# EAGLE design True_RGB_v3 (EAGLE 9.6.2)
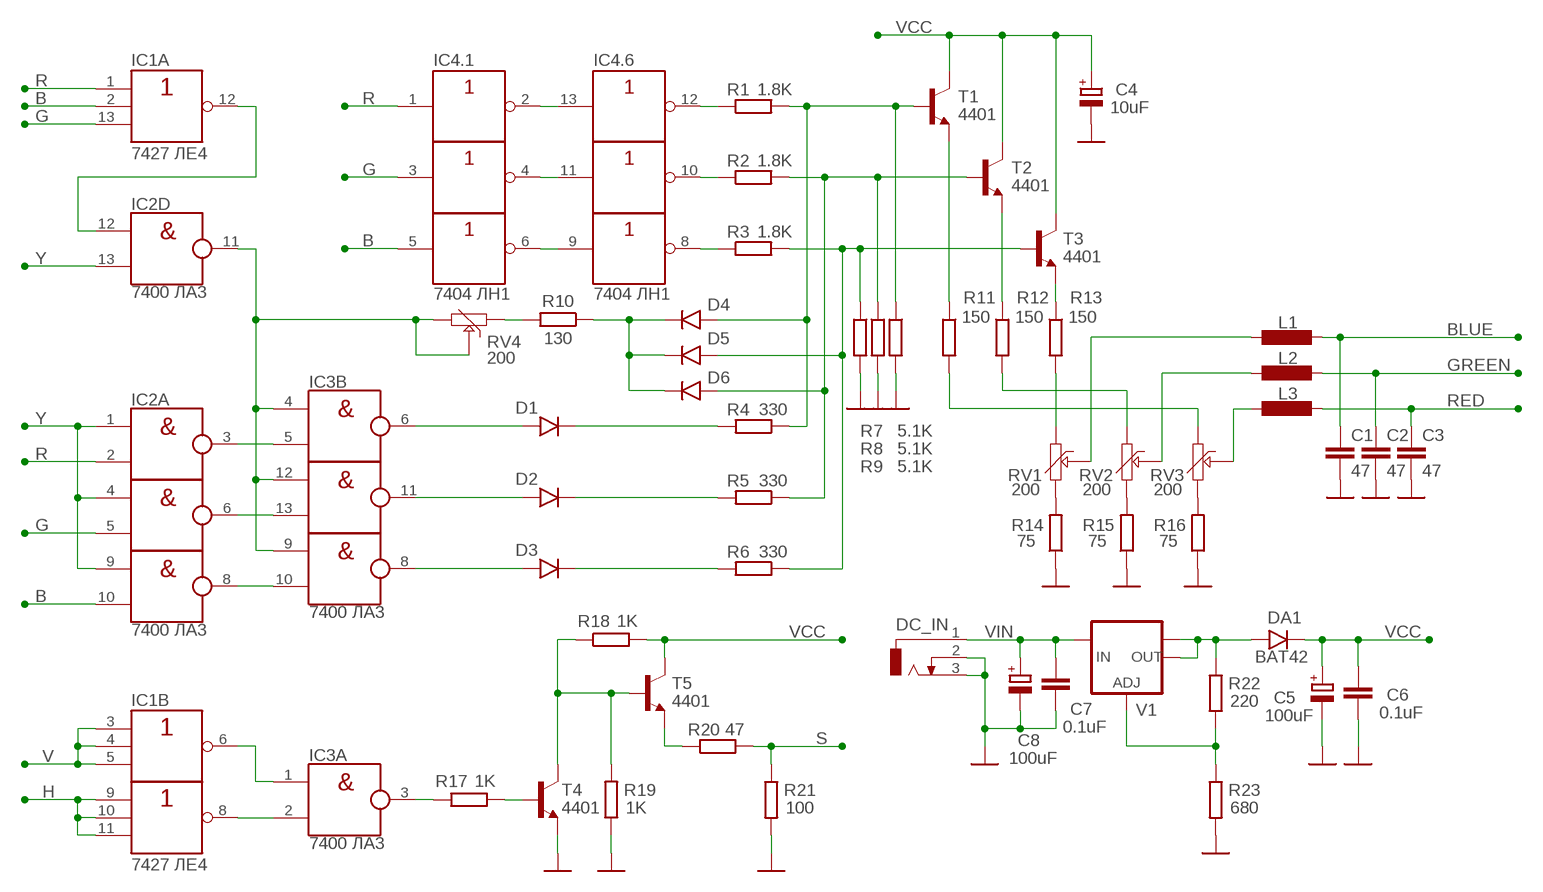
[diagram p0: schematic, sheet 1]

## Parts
C1  47  C-EU050-024X044  [C050-024X044]
C2  47  C-EU050-024X044  [C050-024X044]
C3  47  C-EU050-024X044  [C050-024X044]
C4  10uF  CPOL-EUE2.5-6  [E2,5-6]
C5  100uF  CPOL-EUE2.5-6  [E2,5-6]
C6  0.1uF  C-EU050-024X044  [C050-024X044]
C7  0.1uF  C-EU050-024X044  [C050-024X044]
C8  100uF  CPOL-EUE2.5-6  [E2,5-6]
D1  1N4148AS  [D4148-2]
D2  1N4148AS  [D4148-2]
D3  1N4148AS  [D4148-2]
D4  1N4148AS  [D4148-2]
D5  1N4148AS  [D4148-2]
D6  1N4148AS  [D4148-2]
DA1  BAT42  1N4148AS  [D4148-2]
DC_IN  DCJ0202  [DCJ0202]
IC1  7427 ЛЕ4  74HC27N  [DIL14]
IC2  7400 ЛА3  74HC00N  [DIL14]
IC3  7400 ЛА3  74HC00N  [DIL14]
IC4  7404 ЛН1  74HC04N  [DIL14]
L1  0.56uH  L-EU0207/2V  [0207/2V]
L2  0.56uH  L-EU0207/2V  [0207/2V]
L3  0.56uH  L-EU0207/2V  [0207/2V]
R1  1.8K  R-EU_0207/2V  [0207/2V]
R2  1.8K  R-EU_0207/2V  [0207/2V]
R3  1.8K  R-EU_0207/2V  [0207/2V]
R4  330  R-EU_0207/2V  [0207/2V]
R5  330  R-EU_0207/2V  [0207/2V]
R6  330  R-EU_0207/2V  [0207/2V]
R7  5.1K  R-EU_0207/2V  [0207/2V]
R8  5.1K  R-EU_0207/2V  [0207/2V]
R9  5.1K  R-EU_0207/2V  [0207/2V]
R10  130  R-EU_0207/2V  [0207/2V]
R11  150  R-EU_0207/2V  [0207/2V]
R12  150  R-EU_0207/2V  [0207/2V]
R13  150  R-EU_0207/2V  [0207/2V]
R14  75  R-EU_0207/2V  [0207/2V]
R15  75  R-EU_0207/2V  [0207/2V]
R16  75  R-EU_0207/2V  [0207/2V]
R17  1K  R-EU_0207/2V  [0207/2V]
R18  1K  R-EU_0207/2V  [0207/2V]
R19  1K  R-EU_0207/2V  [0207/2V]
R20  47  R-EU_0207/2V  [0207/2V]
R21  100  R-EU_0207/2V  [0207/2V]
R22  220  R-EU_0207/2V  [0207/2V]
R23  680  R-EU_0207/2V  [0207/2V]
RV1  200  TRIM-6MM  [6MM]
RV2  200  TRIM-6MM  [6MM]
RV3  200  TRIM-6MM  [6MM]
RV4  200  TRIM-6MM  [6MM]
T1  4401  2N4401-NPN-TO92-EBC  [TO92-EBC]
T2  4401  2N4401-NPN-TO92-EBC  [TO92-EBC]
T3  4401  2N4401-NPN-TO92-EBC  [TO92-EBC]
T4  4401  2N4401-NPN-TO92-EBC  [TO92-EBC]
T5  4401  2N4401-NPN-TO92-EBC  [TO92-EBC]
V1  LM1117IMPX-ADJ  [SOT223]

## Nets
B: IC1.2(A:I1) IC2.10(C:I1) IC4.5(.3:I)
BLUE: C1.1 L1.1
G: IC1.13(A:I2) IC2.5(B:I1) IC4.3(.2:I)
GND: C1.2 C2.2 C3.2 C4.- C5.- C6.2 C7.2 C8.- DC_IN.2 DC_IN.3 R7.2 R8.2 R9.2 R14.1 R15.1 R16.1 R19.1 R21.2 R23.2 T4.E
GREEN: C2.1 L2.1
H: IC1.9(C:I0) IC1.10(C:I1) IC1.11(C:I2)
N$1: D3.C R6.2
N$2: D2.C R5.2
N$3: D1.C R4.2
N$4: L1.2 RV1.S
N$5: IC1.12(A:O) IC2.12(D:I0)
N$6: IC1.8(C:O) IC3.2(A:I1)
N$7: L2.2 RV2.S
N$8: D5.A R3.2 R6.1 R7.1 T3.B
N$9: D6.A R2.2 R5.1 R8.1 T2.B
N$10: D4.A R1.2 R4.1 R9.1 T1.B
N$11: L3.2 RV3.S
N$12: R14.2 RV1.A
N$13: R15.2 RV2.A
N$14: R16.2 RV3.A
N$15: R11.1 T1.E
N$16: R12.2 RV2.E
N$17: R11.2 RV3.E
N$18: R12.1 T2.E
N$19: IC2.3(A:O) IC3.5(B:I1)
N$20: IC2.6(B:O) IC3.13(D:I1)
N$21: IC2.8(C:O) IC3.10(C:I1)
N$22: D1.A IC3.6(B:O)
N$23: D2.A IC3.11(D:O)
N$24: D3.A IC3.8(C:O)
N$25: IC4.2(.1:O) IC4.13(.6:I)
N$26: IC4.4(.2:O) IC4.11(.5:I)
N$27: IC4.6(.3:O) IC4.9(.4:I)
N$28: IC4.12(.6:O) R1.1
N$29: IC4.10(.5:O) R2.1
N$30: IC4.8(.4:O) R3.1
N$31: IC3.3(A:O) R17.2
N$32: R22.2 R23.1 V1.1(ADJ)
N$33: IC1.6(B:O) IC3.1(A:I0)
N$34: R17.1 T4.B
N$35: DA1.A R22.1 V1.2(OUT) V1.TAB(OUT1)
N$36: D4.C D5.C D6.C R10.1
N$37: R10.2 RV4.E
N$38: IC2.11(D:O) IC3.4(B:I0) IC3.9(C:I0) IC3.12(D:I0) RV4.A RV4.S
N$39: R13.1 T3.E
N$40: R13.2 RV1.E
N$176: R20.1 T5.E
N$177: R18.1 R19.2 T4.C T5.B
R: IC1.1(A:I0) IC2.2(A:I1) IC4.1(.1:I)
RED: C3.1 L3.1
S: R20.2 R21.1
V: IC1.3(B:I0) IC1.4(B:I1) IC1.5(B:I2)
VCC: C4.+ C5.+ C6.1 DA1.C R18.2 T1.C T2.C T3.C T5.C
VIN: C7.1 C8.+ DC_IN.1 V1.3(IN)
Y: IC2.1(A:I0) IC2.4(B:I0) IC2.9(C:I0) IC2.13(D:I1)

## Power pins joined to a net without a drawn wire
GND: IC1.7(P:GND) IC2.7(P:GND) IC3.7(P:GND) IC4.7(P:GND)
VCC: IC1.14(P:VCC) IC2.14(P:VCC) IC3.14(P:VCC) IC4.14(P:VCC)

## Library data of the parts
C1-C3 C6 C7 = rcl:C-EU: CAPACITOR, European symbol; SPICEPREFIX: C
C4 C5 C8 = rcl:CPOL-EU: POLARIZED CAPACITOR, European symbol; SPICEPREFIX: C
D1-D6 DA1 = 27C322:1N4148
DC_IN = power_jack:DCJ0202: DC POWER JACK Source: DCJ0202.pdf; OC_FARNELL: unknown; OC_NEWARK: unknown
IC1 = 74xx-eu:74*27: Triple 3-input NOR gate
IC2 IC3 = 74xx-eu:74*00: Quad 2-input NAND gate
IC4 = 74xx-eu:74*04: Hex INVERTER
L1-L3 = rcl:L-EU: INDUCTOR, European symbol; SPICEPREFIX: L
R1-R23 = rcl:R-EU_: RESISTOR, European symbol; SPICEPREFIX: R
RV1-RV4 = 27C322:TRIM-6MM
T1-T5 = transistor-neu-to92:*-NPN-: NPN Transistror
V1 = lm1117:LM1117IMPX-ADJ

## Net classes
1 power: width 0.66 mm, clearance 0.254 mm

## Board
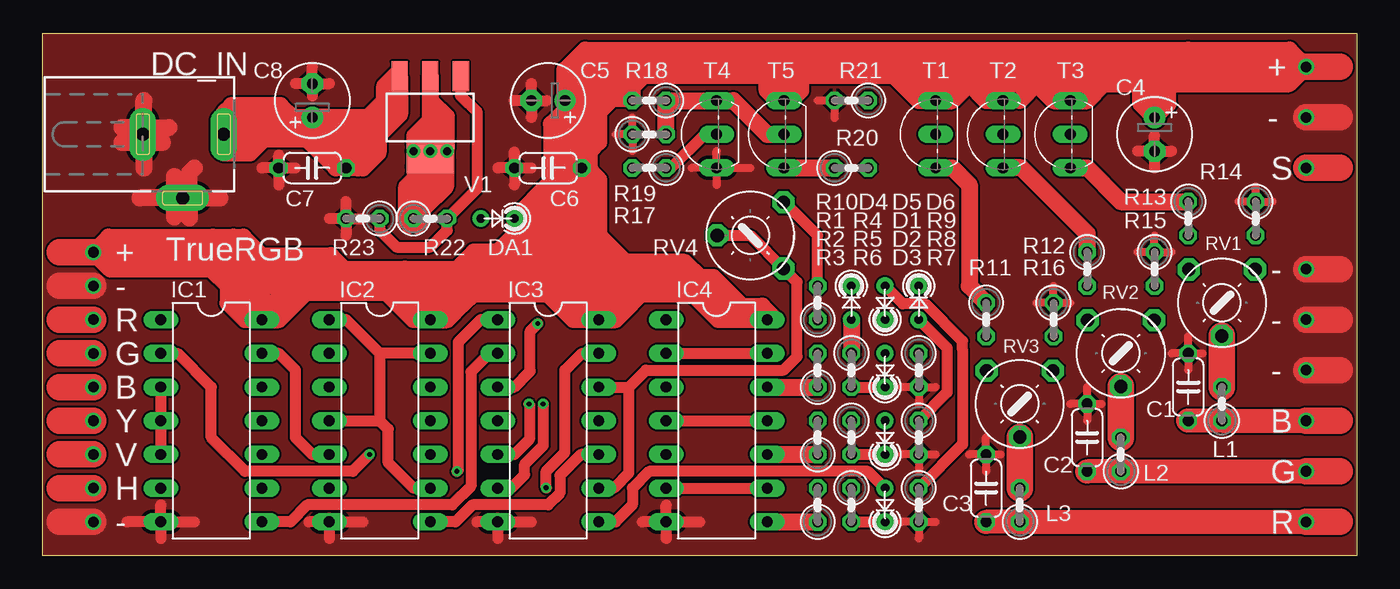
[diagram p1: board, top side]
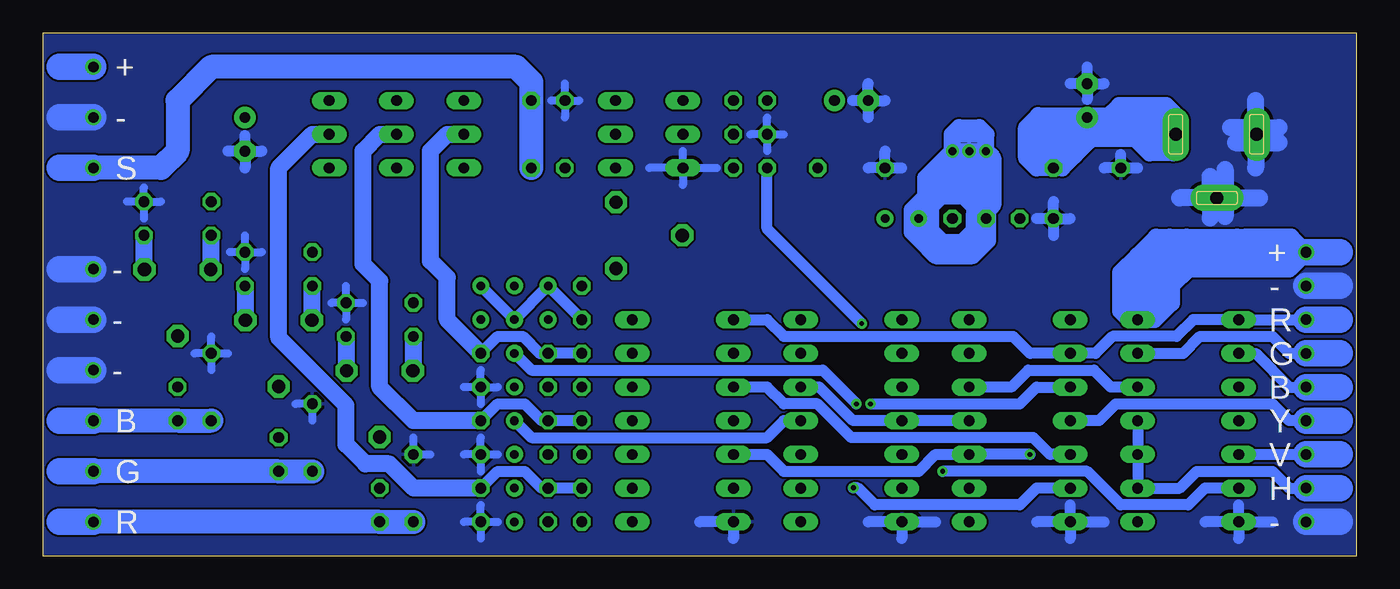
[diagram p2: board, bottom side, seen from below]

Size 99.06 x 39.37 mm. Coordinates in mm from the lower left corner, seen from the top.
Outline: 99.06,39.37 99.06,0 0,0 0,39.37 99.06,39.37
Copper layers (1*16): Top 0.035mm / dielectric 1.5mm / Bottom 0.035mm
Design rules "default *": minimum track width 6mil, minimum drill 0.35mm, track to track 6mil, track to pad 6mil, pad to pad 6mil, via to via 6mil, smd to smd 6mil, copper to edge 2mil, drill to drill 6mil, minimum pad ring 10mil, minimum via ring 8mil, stop-mask expansion 4mil, vias tented up to drill 20mil, thermal gap 10mil

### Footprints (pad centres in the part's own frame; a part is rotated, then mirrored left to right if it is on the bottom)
C050-024X044 = drill 0.813 octagon: 1 -2.54,0; 2 2.54,0
E2,5-6 = drill 0.813 pad 1.6: + -1.27,0 | drill 0.813 pad 1.6 octagon: - 1.27,0
D4148-2 = drill 0.65 pad 1.27: A 1.27,0; C -1.27,0
DCJ0202 = drill 1 pad 2 long: 1 0,3.1; 2 4.8,0; 3 0,-3
DIL14 = drill 0.813 long: 1 -7.62,-3.81; 2 -5.08,-3.81; 3 -2.54,-3.81; 4 0,-3.81; 5 2.54,-3.81; 6 5.08,-3.81; 7 7.62,-3.81; 8 7.62,3.81; 9 5.08,3.81; 10 2.54,3.81; 11 0,3.81; 12 -2.54,3.81; 13 -5.08,3.81; 14 -7.62,3.81
0207/2V = drill 0.813 octagon: 1 -1.27,0; 2 1.27,0
6MM = drill 1 pad 1.676 octagon: A -2.5,-2.5; E 2.5,-2.5; S 0,2.5
TO92-EBC = drill 0.813 long: B 0,-1.27; C 2.54,-1.27; E -2.54,-1.27
SOT223 = smd 1.219 x 2.235: 1 -2.311,-3.099; 2 0,-3.099; 3 2.311,-3.099 | smd 3.6 x 2.2: TAB 0,3.099

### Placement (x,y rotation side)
C1  86.36,12.7 90 top
C2  78.74,8.89 90 top
C3  71.12,5.08 90 top
C4  83.82,31.75 270 top
C5  38.1,34.29 180 top
C6  38.1,29.21 180 top
C7  20.32,29.21 180 top
C8  20.32,34.29 90 top
D1  63.5,13.97 90 top
D2  63.5,8.89 90 top
D3  63.5,3.81 90 top
D4  60.96,19.05 270 top
D5  63.5,19.05 90 top
D6  66.04,19.05 270 top
DA1  34.29,25.4 180 top
DC_IN  10.54,31.75 270 top
IC1  12.7,10.16 270 top
IC2  25.4,10.16 270 top
IC3  38.1,10.16 270 top
IC4  50.8,10.16 270 top
L1  88.9,11.43 90 top
L2  81.28,7.62 90 top
L3  73.66,3.81 90 top
R1  58.42,13.97 90 top
R2  58.42,8.89 90 top
R3  58.42,3.81 90 top
R4  60.96,13.97 270 top
R5  60.96,8.89 270 top
R6  60.96,3.81 270 top
R7  66.04,3.81 270 top
R8  66.04,8.89 270 top
R9  66.04,13.97 270 top
R10  58.42,19.05 90 top
R11  71.12,17.78 270 top
R12  78.74,21.59 270 top
R13  86.36,25.4 270 top
R14  91.44,25.4 270 top
R15  83.82,21.59 270 top
R16  76.2,17.78 270 top
R17  45.72,29.21 180 top
R18  45.72,34.29 180 top
R19  45.72,31.75 0 top
R20  60.96,29.21 0 top
R21  60.96,34.29 180 top
R22  29.21,25.4 0 top
R23  24.13,25.4 180 top
RV1  88.9,19.05 180 top
RV2  81.28,15.24 180 top
RV3  73.66,11.43 180 top
RV4  53.34,24.13 90 top
T1  66.04,31.75 90 top
T2  71.12,31.75 90 top
T3  76.2,31.75 90 top
T4  49.53,31.75 90 top
T5  54.61,31.75 90 top
V1  29.21,33.02 180 top

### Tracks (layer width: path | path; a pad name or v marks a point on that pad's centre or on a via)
B  (via drill 0.35, 0.8)
  Top 0.813: IC1.2 10.16,15.24 12.7,12.7 12.7,8.89 15.24,6.35 23.37,6.35 v24.64,7.62
  Top 2: v3.81,12.7 1.27,12.7
  Bottom 0.813: v24.64,7.62 IC2.10 31.75,7.62 33.02,6.35 43.18,6.35 44.45,7.62 IC4.5 | IC1.2 7.62,15.24 5.08,12.7 v3.81,12.7
  Bottom 2: 1.27,12.7 v3.81,12.7
BLUE  (via drill 0.8)
  Top 1.8: v95.25,10.16 L1.1 C1.1
  Top 2: v95.25,10.16 97.79,10.16
  Bottom 1.8: v95.25,10.16 L1.1 C1.1
  Bottom 2: v95.25,10.16 97.79,10.16
G  (via drill 0.8)
  Top 0.813: IC2.5 20.32,7.62 19.05,8.89 19.05,13.97 17.78,15.24 IC1.13
  Top 2: v3.81,15.24 1.27,15.24
  Bottom 0.813: IC2.5 23.11,7.62 24.38,8.89 38.1,8.89 40.64,11.43 43.18,11.43 44.45,12.7 IC4.3 | IC1.13 13.08,15.24 11.81,16.51 6.35,16.51 5.08,15.24 v3.81,15.24
  Bottom 2: 1.27,15.24 v3.81,15.24
GND  (via drill 0.8)
  Top 0.61: R14.1 92.71,26.67 | R14.1 91.44,27.81 | R14.1 90.17,26.67 | R14.1 91.44,25.4 | R15.1 83.82,24.13 | R15.1 85.09,22.86 | R15.1 82.55,22.86 | R15.1 83.82,21.59 | C1.2 86.36,16.51 | C1.2 85.09,15.24 | C1.2 86.36,13.97 | C1.2 87.44,15.24 | R16.1 76.2,20.32 | R16.1 76.2,17.78 | R16.1 74.93,19.05 | R16.1 77.47,19.05 | R9.2 67.31,12.7 | R9.2 66.04,13.97 | R9.2 64.77,12.7 | R9.2 66.04,11.43 | R8.2 67.31,7.62 | R8.2 66.04,8.89 | R8.2 64.77,7.62 | R8.2 66.04,6.35 | R7.2 67.31,2.54 | R7.2 66.04,3.81 | R7.2 64.77,2.54 | R7.2 66.04,1.27 | C3.2 71.12,8.89 | C3.2 71.12,6.35 | C3.2 69.85,7.62 | C3.2 72.2,7.62 | C2.2 78.74,10.16 | C2.2 78.74,12.7 | C2.2 79.82,11.43 | C2.2 77.47,11.43 | T4.E 50.8,27.94 | T4.E 48.92,29.21 | T4.E 53.34,29.21 | T4.E 50.8,30.48 | R21.2 59.69,32.97 | R21.2 58.42,34.29 | R21.2 60.96,34.29 | R19.1 43.18,31.75 | R19.1 44.45,33.02 | R19.1 44.45,30.48 | R19.1 45.72,31.75
  Top 0.813: C5.- 36.83,35.56 | C5.- 35.56,34.29 | C5.- 38.01,34.29 | C5.- 36.83,33.02 | C6.2 35.56,30.43 | C6.2 34.29,29.21 | C6.2 36.83,29.21 | C6.2 35.56,27.94 | C8.- 20.32,36.83 | C8.- 21.59,35.56 | C8.- 19.05,35.56 | C8.- 20.32,34.63 | C7.2 19.05,29.21 | C7.2 16.51,29.21 | C7.2 17.78,30.18 | C7.2 17.78,27.94 | IC1.7 11.43,2.54 | IC1.7 6.35,2.54 | IC1.7 8.89,3.81 | IC1.7 8.89,1.27 | IC2.7 20.07,2.54 | IC2.7 24.13,2.54 | IC2.7 21.59,1.27 | IC3.7 32.73,2.54 | IC3.7 36.83,2.54 | IC3.7 34.29,1.27 | IC4.7 45.21,2.54 | IC4.7 46.99,3.81 | IC4.7 46.99,1.27 | IC4.7 49.53,2.54 | C4.- 83.82,31.66 | C4.- 83.82,29.21 | C4.- 85.09,30.48 | C4.- 82.55,30.48 | R23.2 22.86,26.67 | R23.2 21.59,25.4 | R23.2 24.13,25.4 | R23.2 22.86,24.13
  Top 1.27: DC_IN.3 8.18,31.11 9.02,31.11 | DC_IN.3 6.91,31.11 5.97,31.11 | DC_IN.3 7.62,31.83 7.62,34.29 | DC_IN.3 7.62,31.67 7.62,29.21 | 9.91,28.57 9.91,27.59 DC_IN.2 | DC_IN.2 9.91,26.32 9.91,25.53 | DC_IN.2 7.34,26.95 | DC_IN.2 13.36,26.95 | DC_IN.2 11.05,27.46 11.05,28.83 11.43,29.21 | DC_IN.2 11.05,26.44 11.05,25.43 | DC_IN.3 7.03,32.26 5.97,32.26 | DC_IN.3 8.05,32.26 9.53,32.26
  Top 2: v3.81,2.54 1.27,2.54 | v95.25,21.59 97.79,21.59 | v95.25,17.78 97.79,17.78 | v95.25,13.97 97.79,13.97 | v95.25,33.02 97.79,33.02 | v3.81,20.32 1.27,20.32
  Bottom 0.61: R19.1 44.45,33.02 | R19.1 43.18,31.75 | R19.1 45.72,31.75 | R19.1 44.45,30.48 | T4.E 48.26,29.21 | T4.E 50.8,30.48 | T4.E 50.8,27.94 | T4.E 53.34,29.21 | R21.2 60.71,34.29 | R21.2 59.69,33.02 | R21.2 58.61,34.29 | R21.2 59.69,35.56 | 78.74,10.16 C2.2 80.01,11.43 | C1.2 86.36,16.51 | C1.2 85.09,15.24 | C1.2 87.63,15.24 | C1.2 86.36,13.97 | 71.12,8.89 C3.2 69.85,7.62 | R8.2 66.04,8.89 | R8.2 64.77,7.62 | R8.2 67.31,7.62 | R8.2 66.04,6.35 | R7.2 66.04,1.27 | R7.2 67.31,2.54 | R7.2 64.77,2.54 | R7.2 66.04,3.81 | R9.2 66.04,13.97 | R9.2 67.31,12.7 | R9.2 64.77,12.7 | R9.2 66.04,11.43 | R16.1 76.2,20.32 | R16.1 74.93,19.05 | R16.1 76.2,17.78 | R16.1 77.32,19.05 | R15.1 83.82,24.13 | R15.1 83.82,21.59 | R15.1 84.94,22.86 | R15.1 82.55,22.86 | R14.1 91.44,27.75 | R14.1 92.71,26.67 | R14.1 90.17,26.67 | R14.1 91.44,25.4
  Bottom 0.813: C7.2 17.78,30.23 | C7.2 19.05,29.21 | C7.2 16.51,29.21 | C8.- 20.32,36.83 | C8.- 20.32,34.38 | C8.- 21.59,35.56 | C8.- 19.05,35.56 | C6.2 34.29,29.21 | C6.2 36.83,29.21 | C6.2 35.56,30.48 | C5.- 36.83,35.56 | C5.- 38.01,34.29 | C5.- 35.56,34.29 | C5.- 36.83,33.02 | C4.- 82.55,30.48 | C4.- 83.82,29.21 | C4.- 85.09,30.48 | C4.- 83.82,31.66 | IC1.7 11.43,2.54 | IC1.7 8.89,3.81 | IC1.7 8.89,1.27 | IC2.7 19.05,2.54 | IC2.7 21.59,3.81 | IC2.7 21.59,1.27 | IC2.7 24.13,2.54 | IC3.7 31.75,2.54 | IC3.7 36.83,2.54 | IC3.7 34.29,1.27 | 49.53,2.54 IC4.7 46.99,1.27 | IC1.7 6.35,2.54 | R23.2 21.59,25.4 | R23.2 22.86,26.67 | R23.2 22.86,24.13 | R23.2 24.13,25.4
  Bottom 1.27: DC_IN.3 7.62,31.83 7.62,34.29 | DC_IN.3 7.62,31.67 7.62,29.21 | DC_IN.3 8.18,31.11 9.14,31.11 | DC_IN.3 6.91,31.11 5.84,31.11 | DC_IN.2 7.34,26.95 | DC_IN.2 9.91,27.59 9.91,29.08 | DC_IN.2 9.91,26.32 9.91,25.55 | DC_IN.2 13.36,26.95 | DC_IN.2 11.05,27.46 11.05,28.57 | DC_IN.2 11.05,26.44 11.05,25.43 | DC_IN.3 7.03,32.26 5.84,32.26 | DC_IN.3 8.05,32.26 9.53,32.26
  Bottom 2: v3.81,2.54 1.27,2.54 | v95.25,33.02 97.79,33.02 | v95.25,21.59 97.79,21.59 | v95.25,17.78 97.79,17.78 | v95.25,13.97 97.79,13.97 | v3.81,20.32 1.27,20.32
  pour Bottom: -10.16,49.53 106.68,49.53 106.68,-12.7 -10.16,-12.7
  pour Top: -10.16,49.53 106.68,49.53 106.68,-12.7 -10.16,-12.7
GREEN  (via drill 0.8)
  Top 1.8: v95.25,6.35 L2.1 C2.1
  Top 2: 97.79,6.35 v95.25,6.35
  Bottom 1.8: v95.25,6.35 L2.1 C2.1
  Bottom 2: v95.25,6.35 97.79,6.35
H  (via drill 0.8)
  Top 2: v3.81,5.08 1.27,5.08
  Bottom 0.813: v3.81,5.08 5.08,5.08 6.35,6.35 12.06,6.35 13.34,5.08 IC1.9 IC1.10 IC1.11
  Bottom 2: v3.81,5.08 1.27,5.08
N$1
  Top 0.813: R6.2 D3.C
N$2
  Top 0.813: R5.2 D2.C
N$3
  Top 0.813: R4.2 D1.C
N$4
  Top 2: RV1.S L1.2
N$5
  Bottom 0.813: IC1.12 18.54,12.7 19.81,13.97 24.77,13.97 26.03,12.7 IC2.12
N$6
  Top 0.813: IC3.2 33.68,15.24 32.28,13.84 32.28,5.23 30.86,3.81 19.94,3.81 18.67,2.54 IC1.8
N$7
  Top 2: RV2.S L2.2
N$8
  Top 0.813: R7.1 69.34,8.38 69.34,15.24 69.34,15.49 69.34,16.17 66.53,18.97 64.85,18.97 D5.A
  Bottom 0.813: R3.2 R6.1 61.47,5.08 62.74,6.35 64.77,6.35 R7.1
  Bottom 1.27: R7.1 71.1,5.08 72.93,6.91 74.73,6.91 76.2,8.38 76.2,11.31 81.28,16.39 81.28,29.21 78.74,31.75 T3.B
N$9
  Top 0.813: R8.1 68.17,12.29 68.17,15.65 D6.A
  Bottom 0.813: R2.2 R5.1 61.47,10.16 62.74,11.43 64.77,11.43 R8.1
  Bottom 1.27: R8.1 71.12,10.16 73.66,12.7 73.66,20.7 74.93,21.97 74.93,30.48 73.66,31.75 T2.B
N$10
  Top 1.27: D4.A R4.1
  Bottom 0.813: R1.2 R4.1 61.59,15.24 62.87,16.51 64.77,16.51 R9.1
  Bottom 1.27: R9.1 68.58,17.78 68.58,20.95 69.83,22.2 69.83,30.5 68.58,31.75 T1.B
N$11
  Top 2: RV3.S L3.2
N$12
  Bottom 1.27: R14.2 91.44,21.59 RV1.A
N$13
  Bottom 1.27: R15.2 83.82,17.78 RV2.A
N$14
  Bottom 1.27: R16.2 76.2,13.97 RV3.A
N$15
  Top 1.27: T1.E 68.58,29.21 69.85,27.94 69.85,20.32 R11.1
N$16
  Bottom 1.27: R12.2 78.78,20.28 RV2.E
N$17
  Bottom 1.27: R11.2 71.16,16.47 RV3.E
N$18
  Top 1.27: R12.1 78.74,24.26 73.79,29.21 T2.E
N$19  (via drill 0.35)
  Top 0.813: IC3.5 35.56,7.62 36.69,8.75 36.69,11.39 v36.66,11.43
  Bottom 0.813: v36.66,11.43 25.4,11.43 24.13,12.7 IC2.3
N$20  (via drill 0.35)
  Top 0.813: v37.95,5.11 37.95,6.35 39.37,7.78 39.37,13.97 40.64,15.24 IC3.13
  Bottom 0.813: IC2.6 24.13,5.08 25.4,3.81 36.32,3.81 37.62,5.11 v37.95,5.11
N$21
  Top 0.813: IC3.10 40.58,7.62 38.99,6.03 38.99,4.7 38.1,3.81 32.39,3.81 31.12,2.54 IC2.8
N$22  (via drill 0.35)
  Top 0.813: IC3.6 35.31,5.08 36.32,6.1 36.32,6.89 37.72,8.29 v37.72,11.43
  Bottom 0.813: v37.72,11.43 40.26,13.97 62.23,13.97 D1.A
N$23
  Bottom 0.813: D2.A 62.23,8.89 44.45,8.89 43.18,10.16 IC3.11
N$24
  Top 0.813: D3.A 62.23,6.35 45.72,6.35 44.45,5.08 44.45,3.81 43.18,2.54 IC3.8
N$25
  Top 0.813: IC4.2 IC4.13
N$26
  Top 0.813: IC4.4 IC4.11
N$27
  Top 0.813: IC4.6 IC4.9
N$28
  Top 1.27: IC4.12 R1.1
N$29
  Top 1.27: IC4.10 R2.1
N$30
  Top 1.27: IC4.8 R3.1
N$31  (via drill 0.35)
  Top 0.813: IC3.3 35.56,12.7 36.75,13.89 36.75,16.92 v37.31,17.48
  Bottom 0.813: v37.31,17.48 44.45,24.61 R17.2
N$32
  Top 0.813: V1.1 31.5,36.09 31.5,34.67 32.77,33.4 32.77,27.69 R22.2 30.48,24.51 29.21,23.24 26.67,23.24 25.4,24.51 R23.1
N$33  (via drill 0.35)
  Top 0.813: IC3.1 33.02,17.78 31.32,16.08 31.32,6.45 v31.22,6.35
  Bottom 0.813: IC1.6 11.43,5.08 12.7,3.81 17.78,3.81 20.32,6.35 v31.22,6.35
N$34
  Top 0.813: R17.1 47.37,29.21 49.91,31.75 T4.B
N$35  (via drill 0.6)
  Top 1.27: V1.2 29.21,34.29 | 29.21,34.29 29.21,32.77 | 29.21,32.77 v29.21,30.48 | v29.21,30.48 V1.TAB | V1.TAB 28.07,31.06 28.07,31.62 29.21,32.77 | 29.21,34.29 30.43,33.07 30.43,30.76 29.59,29.92 V1.TAB | v29.21,30.48 28.07,29.34 28.07,28.45 | 28.07,28.45 28.07,26.67 | 28.07,26.67 28.07,25.53 | 27.43,25.4 R22.1 28.07,25.53 | 28.07,28.45 27.43,27.81 27.43,25.4 | 28.07,25.53 29.21,26.67 V1.TAB | V1.TAB 30.35,29.92 30.35,27.81 28.7,26.16 | 28.7,26.16 28.45,25.91 28.45,25.15 28.19,24.89 27.69,24.89 27.43,25.15 27.43,25.4 | 28.07,26.67 28.7,26.67 28.7,26.16
  Bottom 1.27: DA1.A 33.02,26.54 | 32.51,27.05 31.62,27.94 31.62,29.34 | 31.62,29.34 v30.48,30.48 | v30.48,30.48 v29.21,30.48 | v29.21,30.48 v27.94,30.48 | v27.94,30.48 27.43,29.97 27.43,26.42 27.81,26.04 27.81,25.4 | 27.81,25.4 R22.1 | R22.1 28.43,25.4 28.82,25.79 | 30.48,27.1 31.32,27.1 DA1.A | R22.1 27.94,28.83 29.21,30.1 v29.21,30.48 | v29.21,30.48 29.08,30.34 29.08,26.67 | 29.08,26.67 29.08,26.54 29.63,27.1 | 28.82,25.79 28.82,26.42 29.08,26.67 | v30.48,30.48 30.48,27.1 | 30.48,27.1 29.63,27.1 | 29.63,27.1 29.51,27.1 29.72,27.31 29.72,29.97 v29.21,30.48 | v30.48,30.48 30.48,31.75 | 30.48,31.75 29.97,32.26 28.45,32.26 27.94,31.75 | v27.94,30.48 27.94,31.75 | 27.94,31.75 30.48,31.75 | 31.62,29.34 32.51,28.45 32.51,27.05 | 32.51,27.05 33.02,26.54 | DA1.A 32.13,26.29 32.13,24.51 31.24,23.62 29.72,23.62 28.82,24.52 28.82,25.79 | 27.81,25.4 27.81,23.75 28.96,22.61 31.75,22.61 33.02,23.88 | DA1.A 33.02,23.88 | 33.02,26.54 33.53,26.04 33.53,24.38 33.02,23.88
N$36
  Bottom 0.813: R10.1 D4.C D5.C D6.C
N$37
  Top 0.813: R10.2 58.42,24.13 55.92,26.63 RV4.E
N$38
  Top 0.813: IC3.9 43.05,5.08 44.2,6.22 44.2,12.7 | IC3.12 44.2,12.7 | 44.2,12.7 45.47,13.97 55.85,13.97 56.87,14.99 56.87,20.6 RV4.A 53.34,24.13 RV4.S
  Bottom 0.813: IC3.12 40.51,12.7 37.97,10.16 IC3.4 IC2.11
N$39
  Top 1.27: T3.E 78.74,29.21 81.28,26.67 R13.1
N$40
  Bottom 1.27: R13.2 86.4,24.09 RV1.E
N$176
  Top 1.27: T5.E R20.1
N$177
  Top 1.27: T5.B 54.61,31.75 52.07,34.29 T4.C R18.1 R19.2
R  (via drill 0.8)
  Top 2: v3.81,17.78 1.27,17.78
  Bottom 0.813: IC4.1 44.45,17.78 43.18,16.51 25.91,16.51 24.64,15.24 IC2.2 19.69,15.24 18.42,16.51 13.59,16.51 12.32,17.78 IC1.1 v3.81,17.78
  Bottom 2: 1.27,17.78 v3.81,17.78
RED  (via drill 0.8)
  Top 1.8: v95.25,2.54 L3.1 C3.1
  Top 2: v95.25,2.54 97.79,2.54
  Bottom 1.8: v95.25,2.54 L3.1 C3.1
  Bottom 2: 97.79,2.54 v95.25,2.54
S  (via drill 0.8)
  Top 2: 97.79,29.21 v95.25,29.21
  Bottom 1.8: R20.2 R21.1 62.23,35.69 63.37,36.83 86.36,36.83 88.9,34.29 88.9,30.48 90.17,29.21 v95.25,29.21
  Bottom 2: v95.25,29.21 97.79,29.21
V  (via drill 0.8)
  Top 0.813: IC1.3 IC1.4 IC1.5
  Top 2: v3.81,7.62 1.27,7.62
  Bottom 0.813: IC1.5 v3.81,7.62
  Bottom 2: v3.81,7.62 1.27,7.62
VCC  (via drill 0.8)
  Top 1.27: 31.62,18.92 32.39,19.68 38.1,19.68 | 31.62,18.92 30.48,17.78 IC2.14 27.94,17.78 25.91,19.81 19.81,19.81 | 52.07,17.78 50.16,19.68 49.02,19.68 | 52.07,17.78 IC4.14 55.25,17.78 54.23,18.8 52.71,18.8 50.55,20.95 49.53,20.95 | 18.67,20.32 20.32,20.32 | 18.67,20.32 16.51,20.32 | 27.43,19.68 26.54,20.57 20.57,20.57 20.32,20.32 | 27.43,19.68 30.86,19.68 32.13,20.95 36.83,20.95 | 44.45,36.83 82.8,36.83 | 82.8,36.83 84.84,36.83 | 84.84,36.83 86.36,36.83 | 44.45,36.83 44.45,37.08 40.89,37.08 40.01,36.2 | 44.45,36.83 44.45,35.56 | 44.45,35.56 44.69,35.56 45.32,36.2 54.61,36.2 | 54.61,36.2 55.88,36.2 | 55.88,36.2 57.15,36.2 | 57.15,36.2 64.14,36.2 | 64.14,36.2 64.77,36.2 65.41,35.56 69.85,35.56 | T5.C 55.88,36.2 | T5.C 56.39,34.29 57.15,35.05 57.15,36.2 | T5.C 55.37,34.29 54.61,35.05 54.61,36.2 | 39.37,33.53 C5.+ 39.37,35.56 | 40.51,34.29 40.51,35.81 | 39.37,35.56 39.37,36.58 40.88,38.09 86.36,38.09 | 40.01,36.2 39.37,35.56 | 40.51,34.29 40.26,34.04 40.26,29.59 C6.1 | 40.51,34.29 41.21,34.99 | 44.45,35.56 41.21,35.56 41.21,34.99 | 39.5,29.21 39.37,29.21 39.37,33.53 | 39.5,29.21 C6.1 | 40.01,36.2 41.91,36.2 | 41.91,36.2 43.82,36.2 44.45,36.83 | 39.37,33.53 38.35,32.51 38.35,28.19 | C6.1 40.51,29.34 | C6.1 41.21,29.21 41.21,30.48 | 41.21,30.48 41.21,34.99 | 36.83,20.95 38.48,20.95 | 38.48,20.95 40.64,20.95 | 40.64,20.95 43.18,20.95 | 43.18,20.95 49.53,20.95 | 49.02,19.68 44.45,19.68 | 44.45,19.68 38.1,19.68 | 40.64,23.11 40.64,20.95 | C6.1 41.02,29.21 41.91,28.32 41.91,24.13 | 41.91,24.13 41.91,22.86 | 41.91,22.86 41.91,20.32 | 16.51,20.32 15.24,20.32 | 15.24,20.32 14.99,20.32 | 31.75,22.1 30.23,20.57 28.07,20.57 27.69,20.95 27.94,20.95 27.31,21.59
  Top 1.27: 49.53,20.95 48.39,22.1 43.94,22.1 41.91,24.13 | 14.99,20.32 13.97,21.34 13.97,19.05 15.24,17.78 IC1.14 | 22.73,21.59 27.31,21.59 | 13.97,21.59 14.61,22.23 | 14.61,22.23 14.86,22.48 15.88,22.48 14.35,24 | T2.C 71.12,34.29 69.85,35.56 | 74.93,35.56 73.66,34.29 | 74.93,35.56 76.2,34.29 T3.C 78.74,34.29 80.01,35.56 | 86.36,35.56 86.36,36.83 | 86.36,36.83 86.36,38.09 | 69.85,35.56 68.58,34.29 T1.C 66.04,34.29 64.14,36.2 | 69.85,35.56 74.93,35.56 | 74.93,35.56 80.01,35.56 | 86.36,38.09 93.99,38.09 v95.25,36.83 93.98,35.56 86.36,35.56 | 86.36,35.56 87.63,36.83 | 12.83,24 14.35,24 | 14.35,24 15.11,24 16.51,22.61 21.72,22.61 22.73,21.59 | 12.83,24 13.97,22.86 | 13.97,22.86 14.61,22.23 | 39.05,18.73 40.01,17.78 IC3.14 43.18,17.78 45.72,20.32 | 39.05,18.73 38.1,19.68 | 44.45,19.68 43.5,18.73 39.05,18.73 | 80.01,35.56 83.82,35.56 | 83.82,35.56 86.36,35.56 | 39.5,25.27 39.5,26.67 | 39.5,26.67 39.5,29.21 | 36.83,20.95 39.62,23.75 39.62,25.4 39.5,25.27 | 38.48,20.95 40.64,23.11 | C6.1 40.64,23.11 | 52.07,17.78 50.93,17.78 49.02,19.68 | 27.31,21.59 31.88,21.59 | IC1.14 16.51,20.32 | IC1.14 17.78,17.78 19.81,19.81 | 19.81,19.81 20.32,20.32 | 15.24,20.32 15.24,19.05 IC1.14 | IC1.14 16.51,18.16 18.67,20.32 | 44.45,35.56 R18.2 44.32,34.42 42.93,34.42 41.91,33.4 | 39.5,25.27 36.32,22.1 31.75,22.1 | 22.73,21.59 22.86,21.46 13.72,21.46 13.59,21.59 12.7,21.59 | 12.7,21.59 5.08,21.59 v3.81,22.86 | 12.7,21.59 13.97,20.32 14.99,20.32 | v3.81,22.86 4.95,24 12.83,24 | 13.97,22.86 v3.81,22.86 | 31.75,22.1 32.51,22.86 34.29,22.86 | 34.29,22.86 35.43,22.86 35.56,22.99 | 27.43,19.68 28.19,18.92 31.62,18.92 | 38.35,28.19 DA1.C 35.56,24.13 | 35.56,24.13 35.56,22.99
  Top 1.27: 35.56,24.13 34.29,22.86 | 38.35,28.19 38.35,26.92 35.56,24.13 | 39.5,26.67 35.81,22.99 35.56,22.99 | 41.91,22.86 43.18,21.59 43.18,20.95 | 41.91,36.2 41.91,33.4 | 41.91,33.4 41.91,31.18 41.21,30.48 | C4.+ 83.82,35.56 | C4.+ 82.8,34.04 82.8,36.83 | C4.+ 84.84,34.04 84.84,36.83
  Top 2: 86.36,36.83 87.63,36.83 v95.25,36.83 97.79,36.83 | 1.27,22.86 v3.81,22.86
  Bottom 1.27: 14.1,24 16,22.1 16.51,22.1 | 14.1,24 12.83,24 | 12.83,24 9.02,24 | 9.02,24 8.38,24 | 16.51,20.32 13.59,23.24 | 13.59,23.24 12.83,24 | 13.59,23.24 9.78,23.24 | 9.78,23.24 9.02,24 | 10.03,22.99 9.78,23.24 | 14.99,20.32 12.45,22.86 v3.81,22.86 | 16.51,20.32 15.88,20.32 | 15.88,20.32 14.99,20.32 | 16.51,20.32 17.02,20.32 17.02,18.29 IC1.14 | 16.51,22.61 15.11,24 14.1,24 | 9.53,22.86 8.38,24 | IC1.14 17.14,17.78 17.78,18.41 17.78,21.34 16.51,22.61 | IC1.14 15.88,17.78 | 15.88,17.78 14.99,18.67 14.99,20.32 | IC1.14 15.88,18.41 15.88,20.32 | v3.81,22.86 4.95,24 8.38,24 | v3.81,22.86 5.08,21.59 12.7,21.59 13.97,20.32 13.97,19.05 15.24,17.78 15.88,17.78 | 16.51,20.32 16.51,22.1 | 16.51,22.1 16.51,22.61
  Bottom 2: v3.81,22.86 1.27,22.86 | v95.25,36.83 97.79,36.83
VIN
  Top 1.27: C7.1 22.86,30.48 | 22.86,30.48 22.86,31.11 | 22.86,31.11 22.86,31.62 22.73,31.75 | 22.86,30.48 23.75,30.48 | C7.1 22.86,29.84 | 23.75,30.48 23.75,29.21 | 22.86,29.72 C7.1 | DC_IN.1 13.64,33.02 | 13.64,33.02 18.8,33.02 | 18.8,33.02 C8.+ 21.46,33.02 | 22.23,32.26 21.46,33.02 | 22.23,32.26 14.15,32.26 DC_IN.1 | 22.86,31.11 21.59,31.11 | 19.94,31.37 21.59,31.37 21.59,31.11 | 19.94,31.37 16.64,31.37 | 16.64,31.37 14.02,31.37 DC_IN.1 | C7.1 21.59,30.48 21.59,31.11 | 18.8,33.02 17.91,33.91 14.22,33.91 13.64,33.33 13.64,33.02 | 19.94,31.37 22.1,29.21 23.75,29.21 | DC_IN.1 13.64,30.35 15.62,30.35 16.64,31.37 | 23.75,29.21 24.13,29.21 25.27,30.35 25.27,31.62 26.9,33.25 V1.3 26.77,36.25 26.64,36.25 25.78,35.38 25.78,34.29 | 23.75,30.48 24.13,30.86 24.13,31.75 | 24.13,31.75 25.4,33.02 | 25.4,33.02 25.78,33.4 25.78,34.29 | 22.23,32.26 22.73,31.75 | 22.73,31.75 24.13,31.75 | 21.46,33.02 24.51,33.02 | 24.51,33.02 25.4,33.02 | 25.78,34.29 24.51,33.02
  Bottom 1.27: DC_IN.1 13.64,33.2 14.35,33.91 17.91,33.91 18.8,33.02 C8.+ | DC_IN.1 13.64,30.55 13.84,30.35 15.62,30.35 16.69,31.42 | 16.69,31.42 20.02,31.42 20.14,31.29 | C7.1 22.23,29.21 21.27,30.16 | 20.14,31.29 21.27,30.16 | C7.1 24.13,29.21 24.89,29.97 24.89,32.26 24,33.15 20.45,33.15 C8.+ | DC_IN.1 15.04,33.15 20.19,33.15 C8.+ | DC_IN.1 14.02,32.13 17.78,32.13 17.91,32.26 23.62,32.26 23.75,32.13 | C7.1 23.88,30.23 | 23.75,32.13 23.88,32 23.88,30.23 | 23.88,30.23 21.34,30.23 21.27,30.16 | 23.75,32.13 22.91,31.29 20.14,31.29 | DC_IN.1 13.97,31.42 16.69,31.42
Y  (via drill 0.8)
  Top 0.813: 25.4,15.24 22.86,17.78 IC2.1 | IC2.9 27.94,5.08 26.03,6.99 26.03,9.53 25.4,10.16 | 25.4,15.24 25.4,10.16 | IC2.4 25.4,10.16 | IC2.13 25.4,15.24
  Top 2: v3.81,10.16 1.27,10.16
  Bottom 0.813: IC2.4 19.43,10.16 18.16,11.43 6.35,11.43 5.08,10.16 v3.81,10.16
  Bottom 2: 1.27,10.16 v3.81,10.16

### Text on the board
tPlace: + | - | S | + | TrueRGB | - | - | R | - | G | - | B | Y | B | V | G | H | - | R
bPlace: + | - | S | + | - | - | R | - | G | - | B | Y | B | V | G | H | - | R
